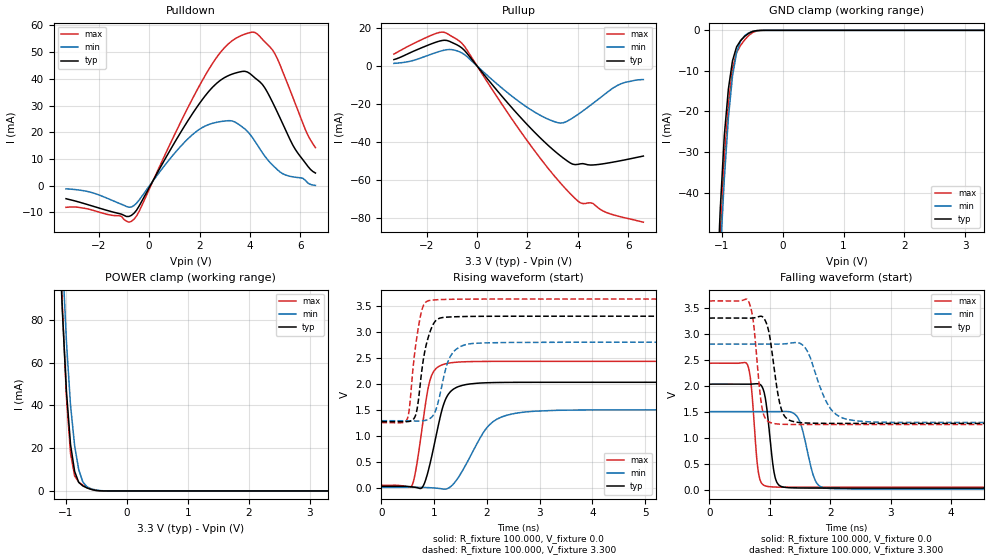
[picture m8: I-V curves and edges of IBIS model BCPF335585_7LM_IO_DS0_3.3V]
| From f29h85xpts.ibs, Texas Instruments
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|   Model BCPF335585_7LM_IO_DS0_3.3V
[Model]   BCPF335585_7LM_IO_DS0_3.3V
Model_type   I/O
Polarity   Non-Inverting
Enable   Active-Low
Vinl =   0.800V
Vinh =   2.000V
Vmeas =  1.650V
Cref =   15.000pF
Vref =   0.0V
|   typ   min   max
C_comp   0.821pF   0.808pF   0.842pF
[Model Spec]
Vinh   2.000V   2.000V   2.000V
Vinl   0.800V   0.800V   0.800V
[Temperature Range]   25   155   -40
[Voltage Range]   3.300V   2.800V   3.630V
[Pullup Reference]   3.300V   2.800V   3.630V
[Pulldown Reference]   0.0V   0.0V   0.0V
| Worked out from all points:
|   slope of the pulldown table from 0 to 0.495 V, typ, clamps not added: 58.5 ohm
|   slope of the pullup table from 0 to 0.495 V, typ, clamps not added: 61 ohm
|   GND clamp passes 1 mA (typ) near -0.58 V on its own axis
|   POWER clamp passes 1 mA (typ) near -0.61 V on its own axis
|   rising waveform, R_fixture 100.000, V_fixture 0.0: 20-80 % time 275ps typ, 516ps min, 211ps max; typ from 0.028 V to 2.03 V
|   rising waveform, R_fixture 100.000, V_fixture 3.300: 20-80 % time 188ps typ, 231ps min, 163ps max; typ from 1.27 V to 3.3 V
|   falling waveform, R_fixture 100.000, V_fixture 0.0: 20-80 % time 115ps typ, 183ps min, 93.9ps max; typ from 2.03 V to 0.028 V
|   falling waveform, R_fixture 100.000, V_fixture 3.300: 20-80 % time 154ps typ, 302ps min, 116ps max; typ from 3.3 V to 1.27 V
[Pulldown]
|Voltage   I(typ)   I(min)   I(max)
-3.3V     -4.863mA   -1.17mA    -8.094mA
-900mV    -11.52mA   -7.773mA   -13.26mA
-600mV    -10.29mA   -7.418mA   -12.51mA
1.1V      17.58mA    13.13mA    20.87mA
2.1V      32.11mA    21.71mA    39.2mA
3.2V      41.43mA    24.35mA    53.53mA
4V        41.96mA    19.25mA    57.31mA
4.5V      37.83mA    12.27mA    54.73mA
5V        29.24mA    6.807mA    49.23mA
5.8V      13.61mA    3.176mA    30.7mA
6.3V      7.235mA    979.6uA    18.91mA
6.6V      4.742mA    97.04uA    14.24mA
[Pullup]
|Voltage   I(typ)   I(min)   I(max)
-3.3V     3.409mA    1.402mA    6.299mA
-1.5V     13.1mA     7.66mA     17.67mA
-800mV    11.18mA    8.014mA    14.07mA
-500mV    8.234mA    6.03mA     10.39mA
1.9V      -29.55mA   -20.94mA   -37.67mA
3.3V      -47.19mA   -30.02mA   -61.46mA
3.8V      -51.69mA   -27.28mA   -68.56mA
4.1V      -51.49mA   -24.59mA   -72mA
4.6V      -52.09mA   -19.65mA   -72.33mA
5V        -51.48mA   -15.54mA   -76.32mA
5.6V      -50.09mA   -10.01mA   -79.03mA
6.6V      -47.39mA   -7.11mA    -82.22mA
[GND_clamp]
|Voltage   I(typ)   I(min)   I(max)
-3.3V     -1.158A    -988.6mA   -1.459A
-1.089V   -68.54mA   -77.63mA   -80.48mA
-1.022V   -44.33mA   -55.86mA   -51.44mA
-955mV    -25.99mA   -36.73mA   -31.56mA
-888mV    -14.45mA   -21.59mA   -18.26mA
-821mV    -7.535mA   -11.36mA   -9.389mA
-754mV    -4.097mA   -5.49mA    -5.516mA
-687mV    -2.502mA   -2.628mA   -3.687mA
-553mV    -723.8uA   -607.5uA   -1.252mA
-419mV    -57.46uA   -69.83uA   -144.1uA
-285mV    -1.004uA   -3.695uA   -2.412uA
3.3V      0A         0A         0A
[POWER_clamp]
|Voltage   I(typ)   I(min)   I(max)
-3.3V     2.015A     2.235A     2.186A
-1.122V   129.6mA    158mA      137.2mA
-1.055V   84.19mA    110mA      86.31mA
-988mV    46.52mA    69.72mA    43.72mA
-921mV    21.67mA    40.06mA    17.56mA
-854mV    9.159mA    21.2mA     7.031mA
-787mV    4.017mA    9.985mA    4.074mA
-720mV    2.344mA    4.225mA    2.739mA
-653mV    1.421mA    1.97mA     1.651mA
-519mV    296.8uA    519.1uA    270.8uA
-318mV    2.374uA    16.61uA    1.127uA
3.3V      0A         0A         0A
[Ramp]
| variable   typ   min   max
dV/dt_r   1.200/0.275n   0.895/0.515n   1.431/0.211n
dV/dt_f   1.216/0.155n   0.906/0.302n   1.426/0.116n
R_load = 100.000
[Rising Waveform]
R_fixture= 100.000
V_fixture= 0.0
V_fixture_min= 0.0
V_fixture_max= 0.0
|time   V(typ)   V(min)   V(max)
0s        28.1mV     8.211mV    45.64mV
586ps     16.78mV    9.135mV    56.43mV
775ps     8.607mV    6.406mV    1.178V
927ps     487.3mV    447.8uV    2.089V
1.126ns   1.412V     -17.76mV   2.353V
1.233ns   1.737V     -22.49mV   2.388V
1.467ns   1.948V     210.9mV    2.417V
2.052ns   2.021V     1.214V     2.43V
2.602ns   2.027V     1.441V     2.431V
10ns      2.028V     1.499V     2.431V
[Rising Waveform]
R_fixture= 100.000
V_fixture= 3.300
V_fixture_min= 2.800
V_fixture_max= 3.630
|time   V(typ)   V(min)   V(max)
0s        1.272V     1.289V     1.251V
488ps     1.271V     1.287V     1.319V
643ps     1.382V     1.284V     2.69V
727ps     1.907V     1.283V     3.236V
799ps     2.493V     1.289V     3.51V
907ps     2.956V     1.323V     3.6V
1.035ns   3.218V     1.506V     3.614V
1.298ns   3.284V     2.508V     3.624V
1.648ns   3.294V     2.764V     3.627V
10ns      3.299V     2.799V     3.628V
[Falling Waveform]
R_fixture= 100.000
V_fixture= 0.0
V_fixture_min= 0.0
V_fixture_max= 0.0
|time   V(typ)   V(min)   V(max)
0s        2.028V     1.499V     2.431V
630ps     2.027V     1.499V     2.402V
691ps     2.028V     1.499V     2.022V
808ps     2.034V     1.499V     354.2mV
953ps     1.536V     1.499V     62.79mV
1.086ns   242.2mV    1.499V     49.18mV
1.265ns   41.27mV    1.502V     46.18mV
1.472ns   30.93mV    1.367V     45.69mV
1.896ns   28.61mV    32.68mV    45.6mV
10ns      28.05mV    8.233mV    45.58mV
[Falling Waveform]
R_fixture= 100.000
V_fixture= 3.300
V_fixture_min= 2.800
V_fixture_max= 3.630
|time   V(typ)   V(min)   V(max)
0s        3.299V     2.799V     3.628V
644ps     3.297V     2.799V     3.629V
734ps     3.302V     2.799V     3.167V
875ps     3.326V     2.799V     1.547V
1.047ns   2.552V     2.798V     1.276V
1.29ns    1.357V     2.808V     1.253V
1.604ns   1.28V      2.694V     1.251V
2.039ns   1.273V     1.506V     1.251V
2.429ns   1.273V     1.321V     1.251V
10ns      1.272V     1.289V     1.251V
